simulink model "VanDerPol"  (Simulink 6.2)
settings: Solver=ode45  StartTime=0.0  StopTime=100  MaxStep=0.05  RelTol=1e-3
libraries: simulink x1

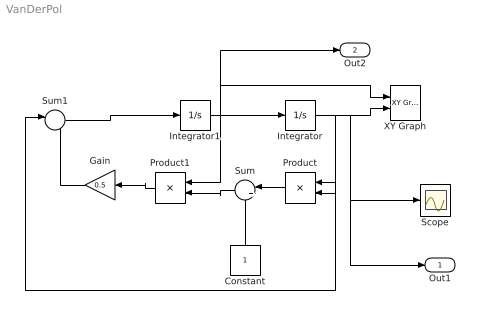
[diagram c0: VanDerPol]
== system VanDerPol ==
  Constant : Constant  Orientation=up
  Gain : Gain  Orientation=left  Gain=0.5
  Integrator : Integrator  InitialCondition=0.1
  Integrator1 : Integrator
  Product : Product  Orientation=left
  Product1 : Product  Orientation=left
  Scope : Scope
  Sum : Sum  Orientation=left  Inputs=|+-
  Sum1 : Sum  Inputs=|--
  XY Graph : simulink/Sinks/XY Graph  xmin=-3  xmax=3  ymin=-3  ymax=3  st=-1
  Out1 : Outport
  Out2 : Outport  Port=2
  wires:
  Integrator/1 -> Product/1, Product/2, Sum1/1, XY Graph/2, Scope/1, Out1/1
  Integrator1/1 -> Product1/1, Integrator/1, XY Graph/1, Out2/1
  Sum/1 -> Product1/2
  Product1/1 -> Gain/1
  Gain/1 -> Sum1/2
  Sum1/1 -> Integrator1/1
  Product/1 -> Sum/1
  Constant/1 -> Sum/2
